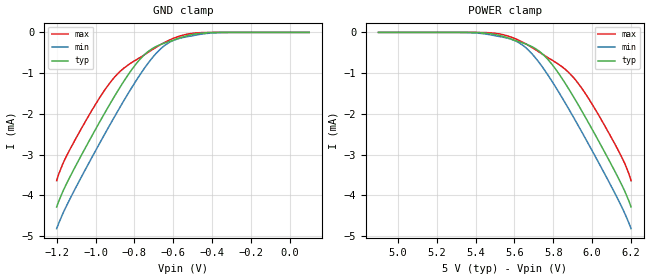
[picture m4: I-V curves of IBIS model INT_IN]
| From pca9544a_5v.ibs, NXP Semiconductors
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[Model]   INT_IN
Model_type Input
Vinh=2.1
Vinl=0.9
C_comp   0.5p   0.5p   0.5p
[Temperature Range] 27   85   -40
[Voltage Range]   5   4.5   5.5
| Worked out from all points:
|   GND clamp passes 1 mA (typ) near -0.83 V on its own axis
[GND Clamp]
-1.2V     -4.288mA   -4.821mA   -3.642mA
-1.17V    -3.927mA   -4.471mA   -3.246mA
-1.11V    -3.352mA   -3.889mA   -2.683mA
-1V       -2.383mA   -2.909mA   -1.767mA
-920mV    -1.713mA   -2.221mA   -1.203mA
-860mV    -1.243mA   -1.724mA   -901.9uA
-770mV    -654.5uA   -1.033mA   -614.4uA
-710mV    -405uA     -638uA     -431uA
-650mV    -271.1uA   -343.2uA   -260.8uA
-540mV    -96.45uA   -116.4uA   -55.76uA
-410mV    -6.277uA   -17.26uA   -938nA
100mV     774fA      7.819pA    302.5fA
[POWER Clamp]
4.9V      774fA      7.819pA    302.5fA
5.41V     -6.277uA   -17.26uA   -938nA
5.54V     -96.45uA   -116.4uA   -55.76uA
5.65V     -271.1uA   -343.2uA   -260.8uA
5.71V     -405uA     -638uA     -431uA
5.77V     -654.5uA   -1.033mA   -614.4uA
5.86V     -1.243mA   -1.724mA   -901.9uA
5.92V     -1.713mA   -2.221mA   -1.203mA
6V        -2.383mA   -2.909mA   -1.767mA
6.11V     -3.352mA   -3.889mA   -2.683mA
6.17V     -3.927mA   -4.471mA   -3.246mA
6.2V      -4.288mA   -4.821mA   -3.642mA
